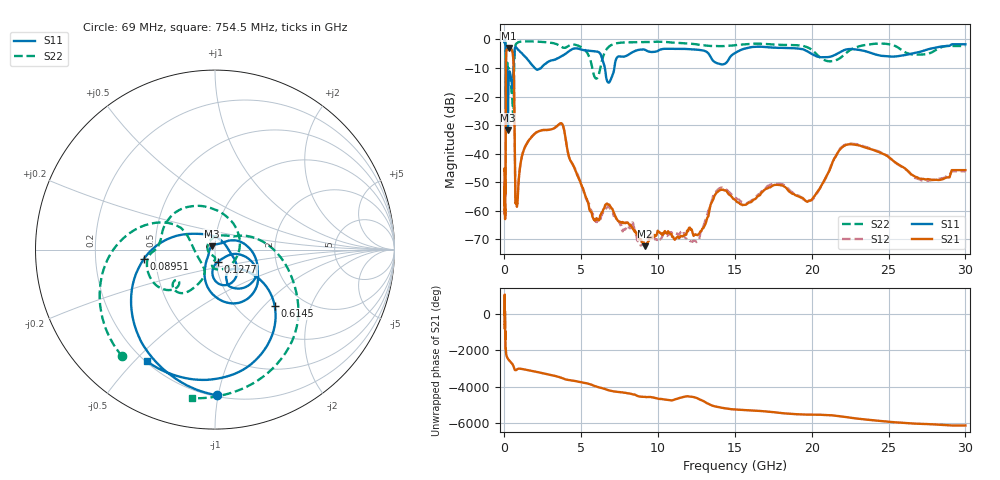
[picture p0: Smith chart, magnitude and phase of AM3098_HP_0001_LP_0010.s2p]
! Date/Time: Thu, Feb 28, 2019 8:31 AM
! Network Analyzer: Agilent Technologies E8364B Rev: A.07.50.67
! Sweep from 0.010 to 30.000 GHz, 1601 Points, Sweep Type: LOG
! Power Supply: 5.022 V, 0.002 A
# Hz S DB R 50
!freq MagS11 AngS11 MagS21 AngS21 MagS12 AngS12 MagS22 AngS22
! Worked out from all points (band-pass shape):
!   1601 points, 10 MHz to 30 GHz, reference 50 ohm
!   highest |S21| = -3.02 dB at 267.8 MHz (marker M1); lowest = -72.5 dB at 9.164 GHz (marker M2)
!   |S21| within 3 dB of the highest: 104.6 MHz to 562.6 MHz (458 MHz wide, 137 % of centre)
!   lowest |S11| = -31.8 dB at 227 MHz (marker M3), VSWR 1.05, Z = 48.3 + j1.88 ohm
!   |S11| at or under -10 dB: 175.6 MHz to 587.8 MHz (412.2 MHz wide, 108 % of centre); 1.969 GHz to 2.38 GHz (410.8 MHz wide, 18.9 % of centre); 6.534 GHz to 7.152 GHz (617.6 MHz wide, 9.03 % of centre)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
!   |S22| runs from -29.0 to -0.5 dB; largest |S21 - S12| = 0.0099
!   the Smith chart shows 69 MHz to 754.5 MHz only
!   S11 on the Smith chart (normalised r, x): 69 MHz: 0.21, -0.99; 89.51 MHz: 0.43, -0.05; 127.7 MHz: 1.02, -0.14; 614.5 MHz: 1.45, -1.16; 754.5 MHz: 0.21, -0.54
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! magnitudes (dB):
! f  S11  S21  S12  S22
! 10 MHz  -0.3  -46.1  -44.8  -0.5
! 38.04 MHz  -0.5  -59.5  -61.2  -0.8
! 69 MHz  -1.8  -50.5  -54.8  -2.1
! 89.51 MHz  -8.0  -18.9  -18.8  -9.6
! 98.93 MHz  -24.2  -7.8  -7.7  -17.2
! 127.7 MHz  -23.1  -4.0  -4.0  -11.2
! 144.7 MHz  -13.4  -3.6  -3.5  -10.2
! 187.7 MHz  -11.7  -3.4  -3.4  -8.3
! 227 MHz  -31.8  -3.1  -3.1  -9.8
! 267.8 MHz  -14.7  -3.0  -3.0  -10.2
! 550.5 MHz  -14.9  -5.4  -5.4  -25.2
! 614.5 MHz  -6.8  -12.6  -12.5  -14.4
! 699.9 MHz  -2.7  -52.8  -52.1  -2.5
! 754.5 MHz  -2.8  -56.8  -57.6  -1.5
! 2.084 GHz  -10.5  -32.6  -32.6  -0.7
! 3.723 GHz  -5.9  -29.4  -29.5  -2.6
! 5.725 GHz  -4.1  -62.1  -60.9  -10.2
! 7.926 GHz  -5.8  -64.2  -66.2  -1.0
! 9.164 GHz  -3.7  -72.5  -72.1  -0.9
! 19.8 GHz  -4.4  -56.5  -56.7  -3.0
! 22.67 GHz  -3.4  -36.8  -36.6  -3.2
! 30 GHz  -1.7  -45.8  -46.3  -2.3
